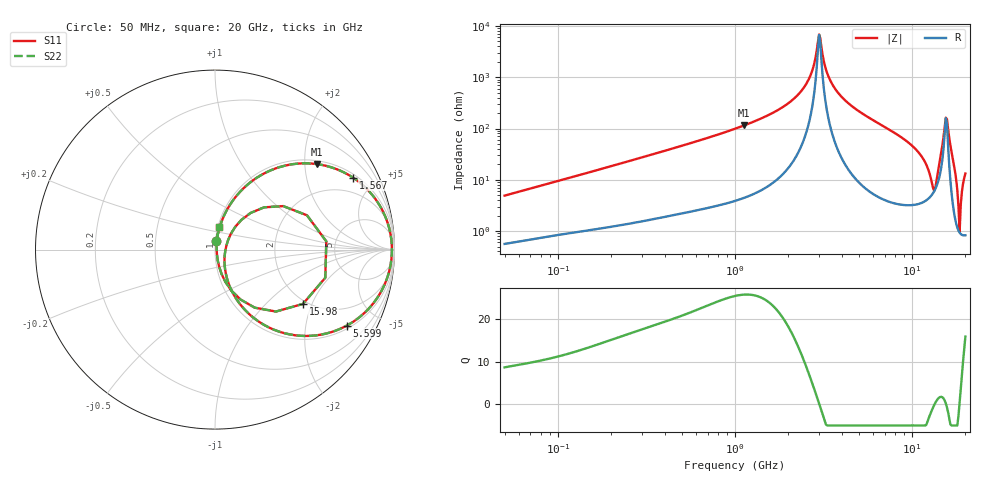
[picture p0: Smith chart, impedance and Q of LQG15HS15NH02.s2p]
!Murata Part Number: LQG15HS15NH02
!These Parameters are Measured in Series Mode Connection
!  o--[Z]--o
!Port1  Port2
!  o-------o
!Freq. Start=50[MHz] Stop=20[GHz], 401[Steps]
# Hz S RI R 50
!Freq.(Hz) S11(Real) S11(Imag) S21(Real) S21(Imag) S12(Real) S12(Imag) S22(Real) S22(Imag)
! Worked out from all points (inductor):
!   401 points, 50 MHz to 20 GHz, reference 50 ohm
!   read as one part in series: L = 15.3 nH near 51.52 MHz
!   highest Q = 25.8 at 1.127 GHz (marker M1), where L = 16.2 nH
!   self-resonance near 2.985 GHz
!   S11 on the Smith chart (normalised r, x): 50 MHz: 1.01, +0.10; 1.567 GHz: 1.16, +3.74; 5.599 GHz: 1.13, -3.38; 15.98 GHz: 1.90, -1.72; 20 GHz: 1.02, +0.26
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5e7  0.00792 0.0481  0.9921 -0.0481  0.9921 -0.0481  0.00792 0.0481
1.364002e8  0.0252 0.1226  0.9748 -0.1226  0.9748 -0.1226  0.0252 0.1226
3.721004e8  0.1163 0.2953  0.8837 -0.2953  0.8837 -0.2953  0.1163 0.2953
1e9  0.4942 0.4807  0.5058 -0.4807  0.5058 -0.4807  0.4942 0.4807
1.127304e9  0.5668 0.4765  0.4332 -0.4765  0.4332 -0.4765  0.5668 0.4765
1.567309e9  0.769 0.4011  0.231 -0.4011  0.231 -0.4011  0.769 0.4011
2.245319e9  0.9372 0.2097  0.0628 -0.2097  0.0628 -0.2097  0.9372 0.2097
2.728004e9  0.9803 0.0709  0.0197 -0.0709  0.0197 -0.0709  0.9803 0.0709
2.940159e9  0.9855 0.0139  0.0145 -0.0139  0.0145 -0.0139  0.9855 0.0139
3.029571e9  0.9857 -0.00918  0.0143 0.00918  0.0143 0.00918  0.9857 -0.00918
3.265178e9  0.9811 -0.0672  0.0189 0.0672  0.0189 0.0672  0.9811 -0.0672
3.626126e9  0.9627 -0.1481  0.0373 0.1481  0.0373 0.1481  0.9627 -0.1481
5.598765e9  0.7333 -0.424  0.2667 0.424  0.2667 0.424  0.7333 -0.424
7.442007e9  0.4737 -0.4801  0.5263 0.4801  0.5263 0.4801  0.4737 -0.4801
1.082228e10  0.131 -0.2925  0.869 0.2925  0.869 0.2925  0.131 -0.2925
1.334722e10  0.057 -0.00782  0.943 0.00782  0.943 0.00782  0.057 -0.00782
1.482269e10  0.2735 0.2355  0.7265 -0.2355  0.7265 -0.2355  0.2735 0.2355
1.550395e10  0.6202 0.046  0.3798 -0.046  0.3798 -0.046  0.6202 0.046
1.597544e10  0.4901 -0.3025  0.5099 0.3025  0.5099 0.3025  0.4901 -0.3025
1.696185e10  0.0909 -0.228  0.9091 0.228  0.9091 0.228  0.0909 -0.228
1.855685e10  0.00923 0.00315  0.9908 -0.00315  0.9908 -0.00315  0.00923 0.00315
2e10  0.025 0.1278  0.975 -0.1278  0.975 -0.1278  0.025 0.1278
